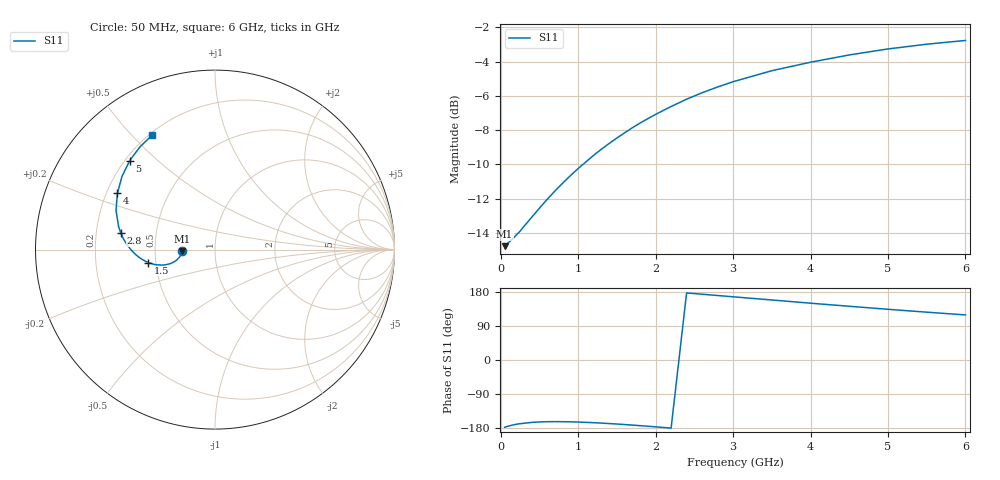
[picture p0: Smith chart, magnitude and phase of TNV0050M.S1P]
! SIEMENS Discrete & RF Semiconductors
! BAS70-07W
! Si Schottky Diode in SOT343
! IF = 50 mA
! S-Parameters:  February  1997
# GHz  S  MA  R  50
!  f  S11
! GHz  MAG  ANG
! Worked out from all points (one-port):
!   34 points, 50 MHz to 6 GHz, reference 50 ohm
!   lowest |S11| = -14.8 dB at 50 MHz (marker M1), VSWR 1.45, Z = 34.6 - j0.593 ohm
!   |S11| at or under -10 dB: start of sweep to 1.061 GHz
!   S11 on the Smith chart (normalised r, x): 50 MHz: 0.69, -0.01; 1.5 GHz: 0.46, -0.08; 2.8 GHz: 0.31, +0.08; 4 GHz: 0.24, +0.25; 5 GHz: 0.22, +0.41; 6 GHz: 0.21, +0.57
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0.05  0.1828 -177.4
0.15  0.1915 -171.8
0.2  0.1969 -169.6
0.25  0.2021 -168.0
0.4  0.2219 -164.7
0.6  0.2503 -162.8
0.7  0.2647 -162.6
0.8  0.279 -162.8
0.9  0.2934 -163.1
1  0.3078 -163.7
1.2  0.3363 -165.4
1.4  0.3641 -167.7
1.5  0.3776 -169.0
1.6  0.3912 -170.3
1.8  0.4177 -173.3
1.9  0.4301 -174.8
2  0.4426 -176.4
2.2  0.4667 -179.7
2.4  0.49 177.0
2.6  0.5118 173.6
2.8  0.5319 170.2
3  0.5511 166.8
3.5  0.5933 158.4
4  0.6281 149.9
4.5  0.6595 141.8
5  0.6866 133.8
5.5  0.7088 126.2
6  0.7269 119.0
